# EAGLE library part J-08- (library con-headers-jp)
HEADER JACK PINS
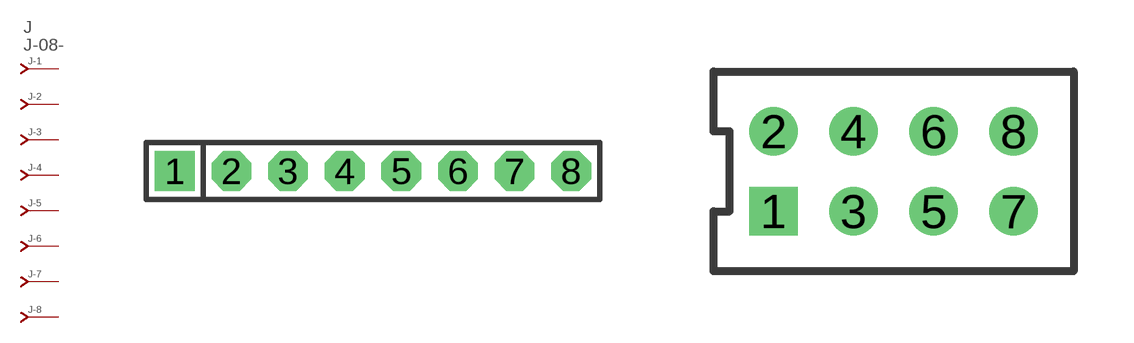
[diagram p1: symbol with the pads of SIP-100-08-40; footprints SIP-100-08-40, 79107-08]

Designator prefix J; gates -2=J-N -3=J-N -4=J-N -5=J-N -6=J-N -7=J-N -8=J-N -1=J-NV

## J-08-SIP-100-40  [SIP-100-08-40]
1  -1:J  pas
2  -2:J  pas
3  -3:J  pas
4  -4:J  pas
5  -5:J  pas
6  -6:J  pas
7  -7:J  pas
8  -8:J  pas

## J-08-79107  [79107-08]
Pads as for SIP-100-08-40

## J-08-79109  [79109-08]
Pads as for SIP-100-08-40

## J-08-87264  [87264-08]
Pads as for SIP-100-08-40

## J-08-87340  [87340-08]
Pads as for SIP-100-08-40

## J-08-100-2X04  [DIL-100-2X04]
Pads as for SIP-100-08-40

## J-08-2MM-2X04  [DIL-2MM-2X04]
Pads as for SIP-100-08-40

## J-08-100-2X04_M  [DIL-100-2X04_M]
Pads as for SIP-100-08-40

## J-08-2MM-2X04_M  [DIL-2MM-2X04_M]
Pads as for SIP-100-08-40

## J-08-535512  [535512-08]
Pads as for SIP-100-08-40

## J-08-SIP-100-32  [SIP-100-08-32]
Pads as for SIP-100-08-40

## J-08-SIP-100-40Y  [SIP-100-08-40Y]
Pads as for SIP-100-08-40

## J-08-SIP-100-32Y  [SIP-100-08-32Y]
Pads as for SIP-100-08-40

## J-08-KK-4455-B08  [KK-4455-B08]
Pads as for SIP-100-08-40

## J-08-KK-4455-A08  [KK-4455-A08]
Pads as for SIP-100-08-40

## J-08-KK-4455-C08  [KK-4455-C08]
Pads as for SIP-100-08-40

## Footprint SIP-100-08-40 (pad centres in mm)
SIP Header - 0.1", 40 mil drill
drill 1.016 pad 1.778 square: 1 -8.89,0
drill 1.016 pad 1.778 octagon: 2 -6.35,0; 3 -3.81,0; 4 -1.27,0; 5 1.27,0; 6 3.81,0; 7 6.35,0; 8 8.89,0

## Footprint 79107-08 (pad centres in mm)
Molex Board-To-Board Receptacal 2.00mm (.079") Pitch Milli-Grid Header, Vertical, Through-Hole Mates with: 87759, 87762, 87758, 87760
drill 0.711 square: 1 -3,-1
drill 0.711: 2 -3,1; 3 -1,-1; 4 -1,1; 5 1,-1; 6 1,1; 7 3,-1; 8 3,1

## Footprint 79109-08 (pad centres in mm)
Molex Board-to-Board Receptacal 2.00mm (.079") Pitch Milli-Grid Header, Vertical, Top/Bottom Entry Mates with: 87758, 87759, 87760, 87831, 87832, 87833
smd 1.12 x 1.83: 1 -3,-2.65; 2 -3,2.65; 3 -1,-2.65; 4 -1,2.65; 5 1,-2.65; 6 1,2.65; 7 3,-2.65; 8 3,2.65
hole 0.914 at -2,0
hole 0.914 at -3,1
hole 0.914 at -3,-1
hole 0.914 at -1,-1
hole 0.914 at -1,1
hole 0.914 at 1,-1
hole 0.914 at 1,1
hole 0.914 at 2,0
hole 0.914 at 3,1
hole 0.914 at 3,-1

## Footprint 87264-08 (pad centres in mm)
Molex Board-To-Board Receptacal 2.00mm (.079") Pitch Milli-Grid Header, Side Entry Mates with 2mm(.079") Mill-Grid Header
drill 0.914 square: 1 -3,-2.25
drill 0.914: 2 -3,2.25; 3 -1,-2.25; 4 -1,2.25; 5 1,-2.25; 6 1,2.25; 7 3,-2.25; 8 3,2.25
